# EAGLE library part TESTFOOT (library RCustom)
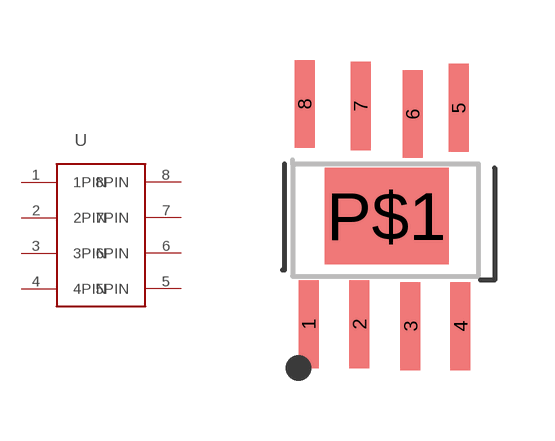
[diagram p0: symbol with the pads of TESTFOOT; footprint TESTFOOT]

Designator prefix -

## TESTFOOT  [TESTFOOT]
1  1PIN
2  2PIN
3  3PIN
4  4PIN  pwr
5  5PIN
6  6PIN
7  7PIN
8  8PIN

## Footprint TESTFOOT (pad centres in mm)
smd 0.5 x 2.2: 1 0,0; 2 1.27,0; 3 2.55,-0.05; 4 3.8,-0.05; 5 3.75,5.4; 6 2.6,5.25; 7 1.3,5.45; 8 -0.1,5.5
smd 3.1 x 2.4: P$1 1.95,2.7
